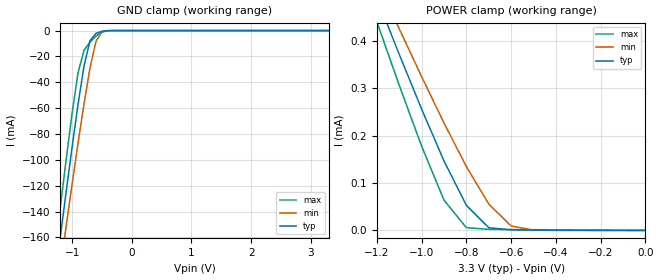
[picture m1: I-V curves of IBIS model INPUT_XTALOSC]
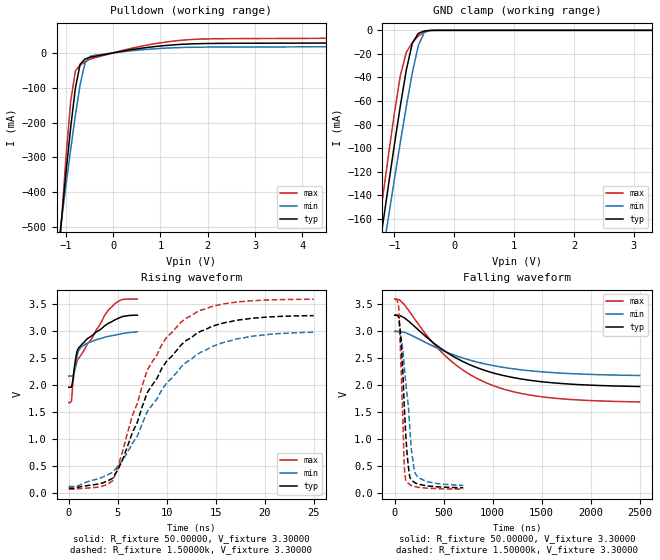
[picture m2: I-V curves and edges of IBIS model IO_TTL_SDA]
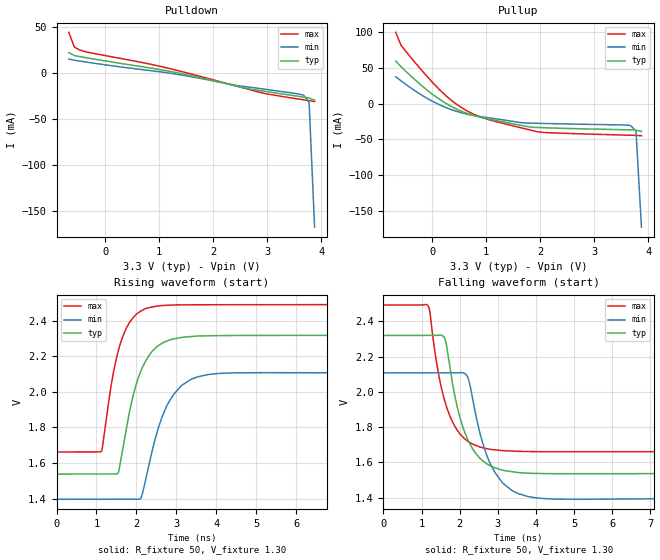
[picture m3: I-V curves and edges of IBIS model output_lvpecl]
[IBIS ver]   4.1
[File name]   5v49ee902.ibs
[File Rev]   2.7
[Date]   July 08, 2013
[Source]   IDT
[Notes]   1. Temp typ=25C, min=85C, max=-40C
[Disclaimer]
READ THESE TERMS AND CONDITIONS CAREFULLY BEFORE USING THIS IBIS MODEL.  BY
USING THIS IBIS MODEL, YOU ARE ACCEPTING AND AGREEING TO THESE TERMS AND
CONDITIONS OF USE.
Integrated Device Technology, Inc. ("IDT") hereby grants the user of this
IBIS model ("User") a non-exclusive, nontransferable license to use this
IBIS model under the following terms: The User is granted this license only
to use the IBIS model for demonstration purposes only and is not granted
rights to sell, copy (except as needed to run the IBIS model), rent, lease
or sub-license (except for demonstration) the IBIS model in whole or in
part, or in modified form to anyone. The User may modify the IBIS model to
suit its specific applications, but  rights to derivative works and such
modifications shall belong to IDT.
THIS IBIS MODEL IS PROVIDED ON AN AS IS" BASIS AND IDT  MAKES ABSOLUTELY NO
WARRANTY WITH RESPECT TO THE INFORMATION CONTAINED HEREIN.  IDT DISCLAIMS
AND USER WAIVES ALL WARRANTIES, EXPRESS AND IMPLIED, INCLUDING WARRANTIES OF
MERCHANTABILITY AND FITNESS FOR A PARTICULAR PURPOSE.  THE ENTIRE RISK AS TO
QUALITY AND PERFORMANCE IS WITH THE USER  ACCORDINGLY, IN NO EVENT SHALL IDT
BE LIABLE FOR ANY DIRECT OR INDIRECT DAMAGES, WHETHER IN CONTRACT OR TORT,
INCLUDING ANY LOST PROFITS OR OTHER INCIDENTAL, CONSEQUENTIAL, EXEMPLARY, OR
PUNITIVE DAMAGES ARISING OUT OF THE USE OR APPLICATION OF THE  IBIS MODEL,
WHETHER OR NOT IDT HAD NOTICE OF SUCH DAMAGES.
IDT reserves the right to make changes without notice to any product herein
to improve reliability, function, or design. IDT does not convey any license
under patent rights or any other intellectual property rights, including
those of third parties. IDT is not obligated to provide  maintenance or
support for the licensed IBIS model.
This model is for  IDT5V49EE902 IDT Programmable Clock
[Copyright]
Copyright 2002, Integrated Device Technology, Inc. All rights  reserved.
|History
|Rev 2.7 Updated on July 08, 2013   add 2v5 model for SE3 and se45 output
|Rev 2.6 Updated on Nov 01, 2012   update out4/4b 5/5b and single end output
|Rev 2.5 Updated on August 07, 2012   update diff table
|Rev 2.4 Updated on August 06, 2012   correct HCSL data error
|Rev 2.3 Updated on August 05, 2012   fix lvmos_1v8_s10 data error
|Rev 2.2 Updated on August 03, 2012   add lvcmos 1v8 output data
|Rev 2.1 Updated on August 02, 2012
|Rev 2.0 Updated on July 27, 2012
|Rev 1.0 Created on May 21, 2009
|   Component IDT5V49EE902
[Component]   IDT5V49EE902
[Manufacturer]   Integrated Device Technology Inc.
[Package]
| Following package parameters are for the 32 pin QFN package
| variable   typ   min   max
R_pkg   72.4655m   58.886m   86.045m
L_pkg   1.47175nH   1.11650nH   1.77850nH
C_pkg   0.07747pF   0.07444pF   0.08050pF
[Pin]  signal_name   model_name
1   VDD   POWER
2   XOUT   NC
3   XIN/REF   INPUT_XTALOSC
4   VDDx   POWER
5   CLKIN   INPUT_TTL
6   GND   GND
7   OUT1   lvcmos_se3
8   OUT2   lvcmos_se3
9   VDD   POWER
10   OUT4   lvcmos_se45
11   OUT4B   lvcmos_se45
12   VDD   POWER
13   GND   GND
14   OUT5   lvcmos_se45
15   OUT5B   lvcmos_se45
16   VDD   POWER
17   GND   GND
18   SDAT   IO_TTL_SDA
19   SCLK   INPUT_TTL
20   CLKSEL   INPUT_TTL
21   AVDD   POWER
22   GND   GND
23   OUT6   lvcmos_se3
24   OUT3   lvcmos_se3
25   VDD   POWER
26   SEL2   INPUT_TTL
27   SEL1   INPUT_TTL
28   SEL0   INPUT_TTL
29   SD/OE   INPUT_TTL
30   OUT0   lvcmos_se3
31   GND   GND
32   VDD   POWER
[Diff Pin]  inv_pin  vdiff   tdelay_typ  tdelay_min  tdelay_max
11   10   0.000V   0.000s   0.000s   0.000s
15   14   0.000V   0.000s   0.000s   0.000s
[Model Selector] output_diff
output_lvds 3.3V LVDS output
output_lvpecl 3.3V LVPECL output
output_hcsl HCSL output
[Model Selector] lvcmos_se3
se3_1v8_s00 slew rate 00
se3_1v8_s01 slew rate 01
se3_1v8_s10 slew rate 10
se3_1v8_s11 slew rate 11
se3_2v5_s00 slew rate 00
se3_2v5_s01 slew rate 01
se3_2v5_s10 slew rate 10
se3_2v5_s11 slew rate 11
se3_3v3_s00 slew rate 00
se3_3v3_s01 slew rate 01
se3_3v3_s10 slew rate 10
se3_3v3_s11 slew rate 11
[Model Selector] lvcmos_se45
se45_1v8_s00 1.8v slew rate 00
se45_1v8_s01 1.8v slew rate 01
se45_1v8_s10 1.8v slew rate 10
se45_1v8_s11 1.8v slew rate 11
se45_2v5_s00 2.5v slew rate 00
se45_2v5_s01 2.5v slew rate 01
se45_2v5_s10 2.5v slew rate 10
se45_2v5_s11 2.5v slew rate 11
se45_3v3_s00 3.3v slew rate 00
se45_3v3_s01 3.3v slew rate 01
se45_3v3_s10 3.3v slew rate 10
se45_3v3_s11 3.3v slew rate 11
| Models and submodels in the file (30): INPUT_XTALOSC (Input), INPUT_TTL (Input), IO_TTL_SDA (I/O_open_drain), output_lvds (Output), output_lvpecl (Output_ECL), output_hcsl (Open_source), se45_1v8_s00 (Output), se45_1v8_s01 (Output), se45_1v8_s10 (Output), se45_1v8_s11 (Output), se45_2v5_s00 (Output), se45_2v5_s01 (Output), se45_2v5_s10 (Output), se45_2v5_s11 (Output), se45_3v3_s00 (Output), se45_3v3_s01 (Output), se45_3v3_s10 (Output), se45_3v3_s11 (Output), se3_1v8_s00 (Output), se3_1v8_s01 (Output), se3_1v8_s10 (Output), se3_1v8_s11 (Output), se3_2v5_s00 (Output), se3_2v5_s01 (Output), se3_2v5_s10 (Output), se3_2v5_s11 (Output), se3_3v3_s00 (Output), se3_3v3_s01 (Output), se3_3v3_s10 (Output), se3_3v3_s11 (Output)
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|   Model INPUT_XTALOSC
[Model]   INPUT_XTALOSC
Model_type   Input
Polarity   Non-Inverting
Vinl =  0.80000V
Vinh =  2.00000V
C_comp   4.00000pF   4.00000pF   4.00000pF
[Temperature Range]   25.00000   100.00000   -40.00000
[Voltage Range]   3.30000V   3.00000V   3.60000V
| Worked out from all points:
|   GND clamp passes 1 mA (typ) near -0.53 V on its own axis
|   POWER clamp passes 1 mA (typ) near -1.62 V on its own axis
[GND_clamp]
| voltage   I(typ)   I(min)   I(max)
-3.3V     -943.7mA   -911.4mA   -977.9mA
-1.3V     -196.5mA   -218.3mA   -176.1mA
-1.2V     -160.4mA   -184.7mA   -137.6mA
-1.1V     -124.9mA   -151.5mA   -99.98mA
-1V       -90.17mA   -118.9mA   -63.99mA
-900mV    -56.99mA   -87.01mA   -32.53mA
-800mV    -27.37mA   -56.54mA   -15.26mA
-700mV    -7.824mA   -28.91mA   -8.942mA
-600mV    -2.175mA   -8.303mA   -4.213mA
-500mV    -492.4uA   -874.3uA   -1.14mA
-400mV    -59.94uA   -63.48uA   -132.1uA
3.3V      67.86nA    72.43nA    13.64nA
[POWER_clamp]
| voltage   I(typ)   I(min)   I(max)
-3.3V     3.118mA    2.794mA    3.419mA
-1.2V     490.8uA    528.9uA    440.7uA
-1.1V     371.9uA    425.9uA    306.6uA
-1V       256.3uA    324.8uA    178uA
-900mV    146.8uA    227uA      63.96uA
-800mV    52.93uA    134.9uA    5.913uA
-700mV    5.782uA    55.77uA    2.388uA
-600mV    1.226uA    9.437uA    1.951uA
-500mV    889.4nA    759.8nA    1.591uA
0V        67.86nA    4.057nA    297.8nA
|   Model IO_TTL_SDA
[Model]   IO_TTL_SDA
Model_type   I/O_open_drain
Polarity   Non-Inverting
Vinl =  0.80000V
Vinh =  2.00000V
Vmeas =  1.65000V
Cref =   5.00pF
Rref =  0.000
Vref =   1.65V
C_comp   3.90000pF   3.90000pF   3.90000pF
[Temperature Range]   25.00000   100.00000   -40.00000
[Voltage Range]   3.30000V   3.00000V   3.60000V
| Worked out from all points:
|   slope of the pulldown table from 0 to 0.495 V, typ, clamps not added: 43.5 ohm
|   GND clamp passes 1 mA (typ) near -0.52 V on its own axis
|   rising waveform, R_fixture 50.00000, V_fixture 3.30000: 20-80 % time 2.7ns typ, 1.89ns min, 3.01ns max; typ from 1.96 V to 3.3 V
|   rising waveform, R_fixture 1.50000k, V_fixture 3.30000: 20-80 % time 5.32ns typ, 6.11ns min, 4.5ns max; typ from 0.084 V to 3.29 V
|   falling waveform, R_fixture 50.00000, V_fixture 3.30000: 20-80 % time 745ns typ, 797ns min, 692ns max; typ from 3.3 V to 1.98 V
|   falling waveform, R_fixture 1.50000k, V_fixture 3.30000: 20-80 % time 55.4ns typ, 83.7ns min, 39.4ns max; typ from 3.3 V to 0.098 V
[Pulldown]
| voltage   I(typ)   I(min)   I(max)
-3.3V     -3.766A    -2.968A    -5.052A
-1.3V     -769.4mA   -703.4mA   -881.9mA
-1V       -344.3mA   -379.3mA   -298.9mA
-900mV    -213.2mA   -275.9mA   -138.2mA
-800mV    -100.1mA   -177.7mA   -51.19mA
-700mV    -32.56mA   -90.56mA   -35.2mA
-600mV    -17.75mA   -30.02mA   -25.79mA
-500mV    -13.24mA   -10.47mA   -18.79mA
600mV     13.4mA     8.771mA    19.31mA
1.5V      24.87mA    15.54mA    36.84mA
5.1V      29.24mA    17.99mA    43.76mA
6.6V      42.47mA    25.45mA    67.13mA
[GND_clamp]
| voltage   I(typ)   I(min)   I(max)
-3.3V     -941mA     -907.6mA   -976.3mA
-1.3V     -202.4mA   -224.6mA   -181.6mA
-1.2V     -166.7mA   -191.4mA   -143.4mA
-1.1V     -131.5mA   -158.6mA   -106mA
-1V       -96.95mA   -126.3mA   -70.13mA
-900mV    -63.73mA   -94.63mA   -38.18mA
-800mV    -33.34mA   -64.12mA   -18.46mA
-700mV    -10.74mA   -35.84mA   -10.48mA
-600mV    -2.575mA   -12.79mA   -4.779mA
-500mV    -539.2uA   -1.691mA   -1.235mA
-400mV    -63.38uA   -109.7uA   -138.9uA
3.3V      1.086nA    4.119nA    592.1pA
[Ramp]
| variable   typ   min   max
dV/dt_r   1.92508/5.19520n   1.72182/6.10290n   2.11914/4.49638n
dV/dt_f   1.92147/55.29974n   1.71552/81.65226n   2.11722/40.58984n
R_load = 1.50000k
[Rising Waveform]
R_fixture = 50.00000
V_fixture = 3.30000
V_fixture_min = 3.00000
V_fixture_max = 3.60000
| Time   typ   min   max
0s        1.96V      2.167V     1.674V
280ps     1.961V     2.167V     1.703V
420ps     2.099V     2.171V     2.041V
560ps     2.318V     2.227V     2.253V
840ps     2.628V     2.535V     2.442V
980ps     2.685V     2.632V     2.491V
1.82ns    2.849V     2.774V     2.737V
3.78ns    3.115V     2.894V     3.327V
5.32ns    3.262V     2.952V     3.581V
7ns       3.299V     2.991V     3.599V
[Rising Waveform]
R_fixture = 1.50000k
V_fixture = 3.30000
V_fixture_min = 3.00000
V_fixture_max = 3.60000
| Time   typ   min   max
0s        83.54mV    113.3mV    64.1mV
4.5ns     268.8mV    380.5mV    223.7mV
5.5ns     615.4mV    601.9mV    769mV
6.5ns     1.121V     917.6mV    1.436V
7ns       1.309V     1.054V     1.66V
8ns       1.855V     1.503V     2.273V
10ns      2.446V     2.04V      2.89V
11.5ns    2.752V     2.344V     3.177V
16ns      3.163V     2.804V     3.515V
25ns      3.292V     2.982V     3.596V
[Falling Waveform]
R_fixture = 50.00000
V_fixture = 3.30000
V_fixture_min = 3.00000
V_fixture_max = 3.60000
| Time   typ   min   max
0s        3.3V       3V         3.6V
50ns      3.296V     2.998V     3.587V
100ns     3.251V     2.982V     3.494V
350ns     2.855V     2.763V     2.874V
550ns     2.588V     2.6V       2.49V
750ns     2.394V     2.475V     2.219V
950ns     2.259V     2.385V     2.034V
1.2us     2.147V     2.308V     1.885V
1.5us     2.066V     2.25V      1.786V
2.5us     1.976V     2.181V     1.69V
[Falling Waveform]
R_fixture = 1.50000k
V_fixture = 3.30000
V_fixture_min = 3.00000
V_fixture_max = 3.60000
| Time   typ   min   max
0s        3.3V       3V         3.6V
42ns      3.262V     2.996V     3.442V
70ns      2.688V     2.847V     2.087V
98ns      1.611V     2.341V     473.4mV
112ns     1.111V     2.056V     243.5mV
140ns     485.4mV    1.603V     179.4mV
154ns     296mV      1.221V     155.3mV
168ns     242.8mV    847.9mV    138.9mV
210ns     186.7mV    363.7mV    115.8mV
700ns     97.55mV    140.8mV    71.3mV
[Model]   output_lvpecl
Model_type   Output_ECL
Polarity   Non-Inverting
|   typ   min   max
C_comp   2pF   1.5pF   2.5pF
Vmeas = 1.95V
Rref = 50
Cref = 0
Vref = 1.3V
|   typ   min   max
[Voltage range]   3.3V   3.135V   3.465V
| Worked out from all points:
|   rising waveform, R_fixture 50, V_fixture 1.30: 20-80 % time 534ps typ, 606ps min, 451ps max; typ from 1.54 V to 2.32 V
|   falling waveform, R_fixture 50, V_fixture 1.30: 20-80 % time 574ps typ, 609ps min, 527ps max; typ from 2.32 V to 1.54 V
[Pulldown]
|Voltage   I (typ)   I (min)   I (max)
|Note, modeling breaks down at 250mA and above.  This is well beyond the functional   |
|operating range of the device.  Should this scenario occur, catastrophic failure and   |
|possible damage to the device and/or board is of higher concern than the I-V curve   |
|behavior.  The IBIS checker will flag currents in excess of 10A with warnings.  Lines   |
|with currents in excess of 0.35 A have been commented out.  The points still remain|
|available to the user if the user desires to use them.   |
|-3.30000e+00   3.30641e+01   2.49914e+01   4.38849e+01
|-3.19898e+00   3.16607e+01   2.38842e+01   4.20980e+01
|-3.09796e+00   3.02581e+01   2.27777e+01   4.03117e+01
|-2.99694e+00   2.88562e+01   2.16720e+01   3.85264e+01
|-2.89592e+00   2.74551e+01   2.05672e+01   3.67423e+01
|-2.79490e+00   2.60551e+01   1.94634e+01   3.49594e+01
|-2.69388e+00   2.46561e+01   1.83607e+01   3.31775e+01
|-2.59286e+00   2.32583e+01   1.72592e+01   3.13966e+01
|-2.49184e+00   2.18620e+01   1.61591e+01   2.96168e+01
|-2.39082e+00   2.04675e+01   1.50607e+01   2.78382e+01
|-2.28980e+00   1.90751e+01   1.39641e+01   2.60611e+01
|-2.18878e+00   1.76846e+01   1.28696e+01   2.42857e+01
|-2.08776e+00   1.62964e+01   1.17779e+01   2.25121e+01
|-1.98673e+00   1.49107e+01   1.06894e+01   2.07407e+01
|-1.88571e+00   1.35280e+01   9.60463e+00   1.89718e+01
|-1.78469e+00   1.21491e+01   8.52420e+00   1.72060e+01
|-1.68367e+00   1.07746e+01   7.44910e+00   1.54439e+01
|-1.58265e+00   9.40591e+00   6.38088e+00   1.36863e+01
|-1.48163e+00   8.04461e+00   5.32189e+00   1.19346e+01
|-1.38061e+00   6.69331e+00   4.27582e+00   1.01904e+01
|-1.27959e+00   5.35620e+00   3.24912e+00   8.45656e+00
|-1.17857e+00   4.04066e+00   2.25420e+00   6.73744e+00
|-1.07755e+00   2.76142e+00   1.31931e+00   5.04113e+00
|-9.76531e-01   1.55427e+00   5.24768e-01   3.38438e+00
|-8.75510e-01   5.35619e-01   9.10535e-02   1.81128e+00
|-7.74490e-01   6.46367e-02   2.16971e-02   4.96338e-01
-673.5mV  22.71mA    15.59mA    44.66mA
-572.4mV  19.44mA    14.32mA    28.67mA
-471.4mV  18.21mA    13.39mA    25.45mA
-370.4mV  17.17mA    12.49mA    23.61mA
1.044V    3.829mA    1.478mA    7.282mA
1.549V    -2.056mA   -3.223mA   -51.59uA
2.357V    -12.83mA   -12.46mA   -12.7mA
2.66V     -16.9mA    -14.93mA   -17.5mA
2.963V    -19.58mA   -17.29mA   -22.04mA
3.67V     -25.75mA   -23.67mA   -28.75mA
3.771V    -26.86mA   -32.04mA   -29.63mA
3.872V    -29.23mA   -167.3mA   -30.63mA
| 3.97347e+00   -3.47071e-02   -1.04797e+00   -3.28632e-02
| 4.07449e+00   -7.42742e-02   -2.67305e+00   -3.86876e-02
| 4.17551e+00   -7.36046e-01   -4.58869e+00   -4.80592e-02
| 4.27653e+00   -2.68947e+00   -6.62812e+00   -6.21080e-02
| 4.37755e+00   -5.16615e+00   -8.73294e+00   -3.32880e-01
| 4.47857e+00   -7.82753e+00   -1.08776e+01   -2.58593e+00
| 4.57959e+00   -1.05770e+01   -1.30488e+01   -6.00998e+00
| 4.68061e+00   -1.33771e+01   -1.52389e+01   -9.74161e+00
| 4.78163e+00   -1.62098e+01   -1.74432e+01   -1.35985e+01
| 4.88265e+00   -1.90653e+01   -1.96585e+01   -1.75220e+01
| 4.98367e+00   -2.19374e+01   -2.18826e+01   -2.14866e+01
| 5.08469e+00   -2.48223e+01   -2.41146e+01   -2.54789e+01
| 5.18571e+00   -2.77173e+01   -2.63531e+01   -2.94912e+01
| 5.28673e+00   -3.06204e+01   -2.85968e+01   -3.35185e+01
| 5.38776e+00   -3.35301e+01   -3.08448e+01   -3.75575e+01
| 5.48878e+00   -3.64456e+01   -3.30966e+01   -4.16060e+01
| 5.58980e+00   -3.93662e+01   -3.53516e+01   -4.56621e+01
| 5.69082e+00   -4.22918e+01   -3.76094e+01   -4.97246e+01
| 5.79184e+00   -4.52214e+01   -3.98697e+01   -5.37926e+01
| 5.89286e+00   -4.81542e+01   -4.21323e+01   -5.78652e+01
| 5.99388e+00   -5.10899e+01   -4.43969e+01   -6.19419e+01
| 6.09490e+00   -5.40281e+01   -4.66634e+01   -6.60221e+01
| 6.19592e+00   -5.69685e+01   -4.89314e+01   -7.01060e+01
| 6.29694e+00   -5.99109e+01   -5.12010e+01   -7.41936e+01
| 6.39796e+00   -6.28552e+01   -5.34719e+01   -7.82839e+01
| 6.49898e+00   -6.58011e+01   -5.57441e+01   -8.23765e+01
| 6.60000e+00   -6.87485e+01   -5.80174e+01   -8.64711e+01
[Pullup]
|Voltage   I (typ)   I (min)   I (max)
|Note, modeling breaks down at 250mA and above.  This is well beyond the functional   |
|operating range of the device.  Should this scenario occur, catastrophic failure and   |
|possible damage to the device and/or board is of higher concern than the I-V curve   |
|behavior.  The IBIS checker will flag currents in excess of 10A with warnings.  Lines   |
|with currents in excess of 0.35 A have been commented out.  The points still remain|
|available to the user if the user desires to use them.   |
|-3.30000e+00   3.30646e+01   2.49917e+01   4.38858e+01
|-3.19898e+00   3.16613e+01   2.38845e+01   4.20992e+01
|-3.09796e+00   3.02586e+01   2.27781e+01   4.03137e+01
|-2.99694e+00   2.88568e+01   2.16724e+01   3.85290e+01
|-2.89592e+00   2.74558e+01   2.05677e+01   3.67452e+01
|-2.79490e+00   2.60558e+01   1.94639e+01   3.49621e+01
|-2.69388e+00   2.46570e+01   1.83612e+01   3.31800e+01
|-2.59286e+00   2.32594e+01   1.72598e+01   3.13989e+01
|-2.49184e+00   2.18635e+01   1.61598e+01   2.96189e+01
|-2.39082e+00   2.04694e+01   1.50614e+01   2.78402e+01
|-2.28980e+00   1.90769e+01   1.39649e+01   2.60629e+01
|-2.18878e+00   1.76863e+01   1.28707e+01   2.42873e+01
|-2.08776e+00   1.62980e+01   1.17792e+01   2.25136e+01
|-1.98673e+00   1.49122e+01   1.06908e+01   2.07421e+01
|-1.88571e+00   1.35295e+01   9.60606e+00   1.89732e+01
|-1.78469e+00   1.21505e+01   8.52558e+00   1.72074e+01
|-1.68367e+00   1.07761e+01   7.45048e+00   1.54454e+01
|-1.58265e+00   9.40743e+00   6.38232e+00   1.36879e+01
|-1.48163e+00   8.04629e+00   5.32346e+00   1.19363e+01
|-1.38061e+00   6.69525e+00   4.27765e+00   1.01924e+01
|-1.27959e+00   5.35855e+00   3.25142e+00   8.45890e+00
|-1.17857e+00   4.04369e+00   2.25736e+00   6.74033e+00
|-1.07755e+00   2.76571e+00   1.32432e+00   5.04491e+00
|-9.76531e-01   1.56136e+00   5.34702e-01   3.38984e+00
|-8.75510e-01   5.51351e-01   1.12022e-01   1.82082e+00
|-7.74490e-01   9.94522e-02   4.65435e-02   5.21672e-01
-673.5mV  59.85mA    37.79mA    99.96mA
-572.4mV  51.65mA    31.85mA    81.49mA
-269.4mV  30.37mA    15.71mA    53.55mA
33.67mV   11.68mA    2.348mA    27.77mA
437.8mV   -6.926mA   -10.31mA   28.84uA
740.8mV   -15.86mA   -16.09mA   -13.68mA
1.044V    -21.4mA    -19.66mA   -22.19mA
1.65V     -30.33mA   -26.55mA   -33.81mA
1.953V    -33.29mA   -27.42mA   -39.29mA
3.67V     -36.6mA    -30.48mA   -44.12mA
3.771V    -37.03mA   -38.18mA   -44.33mA
3.872V    -38.65mA   -172.8mA   -44.69mA
| 3.97347e+00   -4.31075e-02   -1.05342e+00   -4.62337e-02
| 4.07449e+00   -8.15915e-02   -2.67922e+00   -5.10210e-02
| 4.17551e+00   -7.43393e-01   -4.59615e+00   -5.89005e-02
| 4.27653e+00   -2.69724e+00   -6.63718e+00   -7.12793e-02
| 4.37755e+00   -5.17451e+00   -8.74377e+00   -3.41726e-01
| 4.47857e+00   -7.83699e+00   -1.08903e+01   -2.59660e+00
| 4.57959e+00   -1.05880e+01   -1.30634e+01   -6.02150e+00
| 4.68061e+00   -1.33898e+01   -1.52556e+01   -9.75386e+00
| 4.78163e+00   -1.62244e+01   -1.74619e+01   -1.36115e+01
| 4.88265e+00   -1.90818e+01   -1.96793e+01   -1.75361e+01
| 4.98367e+00   -2.19559e+01   -2.19053e+01   -2.15021e+01
| 5.08469e+00   -2.48428e+01   -2.41385e+01   -2.54961e+01
| 5.18571e+00   -2.77398e+01   -2.63776e+01   -2.95102e+01
| 5.28673e+00   -3.06450e+01   -2.86217e+01   -3.35395e+01
| 5.38776e+00   -3.35569e+01   -3.08701e+01   -3.75806e+01
| 5.48878e+00   -3.64744e+01   -3.31221e+01   -4.16311e+01
| 5.58980e+00   -3.93968e+01   -3.53773e+01   -4.56893e+01
| 5.69082e+00   -4.23232e+01   -3.76353e+01   -4.97540e+01
| 5.79184e+00   -4.52533e+01   -3.98959e+01   -5.38241e+01
| 5.89286e+00   -4.81864e+01   -4.21586e+01   -5.78989e+01
| 5.99388e+00   -5.11224e+01   -4.44234e+01   -6.19778e+01
| 6.09490e+00   -5.40609e+01   -4.66900e+01   -6.60602e+01
| 6.19592e+00   -5.70015e+01   -4.89582e+01   -7.01457e+01
| 6.29694e+00   -5.99442e+01   -5.12279e+01   -7.42340e+01
| 6.39796e+00   -6.28887e+01   -5.34990e+01   -7.83248e+01
| 6.49898e+00   -6.58349e+01   -5.57713e+01   -8.24178e+01
| 6.60000e+00   -6.87825e+01   -5.80448e+01   -8.65128e+01
[Ramp]
|   typ   min   max
dV/dt_r   0.467/0.533n   0.426/0.609n   0.497/0.451n
dV/dt_f   0.471/0.575n   0.43/0.619n   0.5/0.528n
R_load =   50.0000
[Rising Waveform]
R_fixture = 50
V_fixture = 1.30   | VCC_typ - 2V
V_fixture_max = 1.465   | VCC_max - 2V
V_fixture_min = 1.135   | VCC_min - 2V
C_fixture = 0.0p
| Time   typ   min   max
0s        1.538V     1.397V     1.663V
1.127ns   1.538V     1.397V     1.667V
1.371ns   1.538V     1.397V     2.041V
1.541ns   1.544V     1.397V     2.227V
1.902ns   1.964V     1.397V     2.413V
2.105ns   2.114V     1.401V     2.453V
2.213ns   2.167V     1.489V     2.467V
2.718ns   2.282V     1.901V     2.486V
3.383ns   2.311V     2.073V     2.489V
10ns      2.318V     2.107V     2.491V
[Falling Waveform]
R_fixture = 50
V_fixture = 1.30   | VCC_typ - 2V
V_fixture_max = 1.465   | VCC_max - 2V
V_fixture_min = 1.135   | VCC_min - 2V
C_fixture = 0.0p
| Time   typ   min   max
0s        2.319V     2.108V     2.492V
1.173ns   2.319V     2.108V     2.487V
1.412ns   2.32V      2.108V     2.143V
1.582ns   2.312V     2.108V     1.97V
1.928ns   1.922V     2.108V     1.786V
2.199ns   1.736V     2.089V     1.722V
2.5ns     1.631V     1.794V     1.69V
2.93ns    1.569V     1.542V     1.671V
3.75ns    1.54V      1.409V     1.662V
10ns      1.537V     1.395V     1.662V
